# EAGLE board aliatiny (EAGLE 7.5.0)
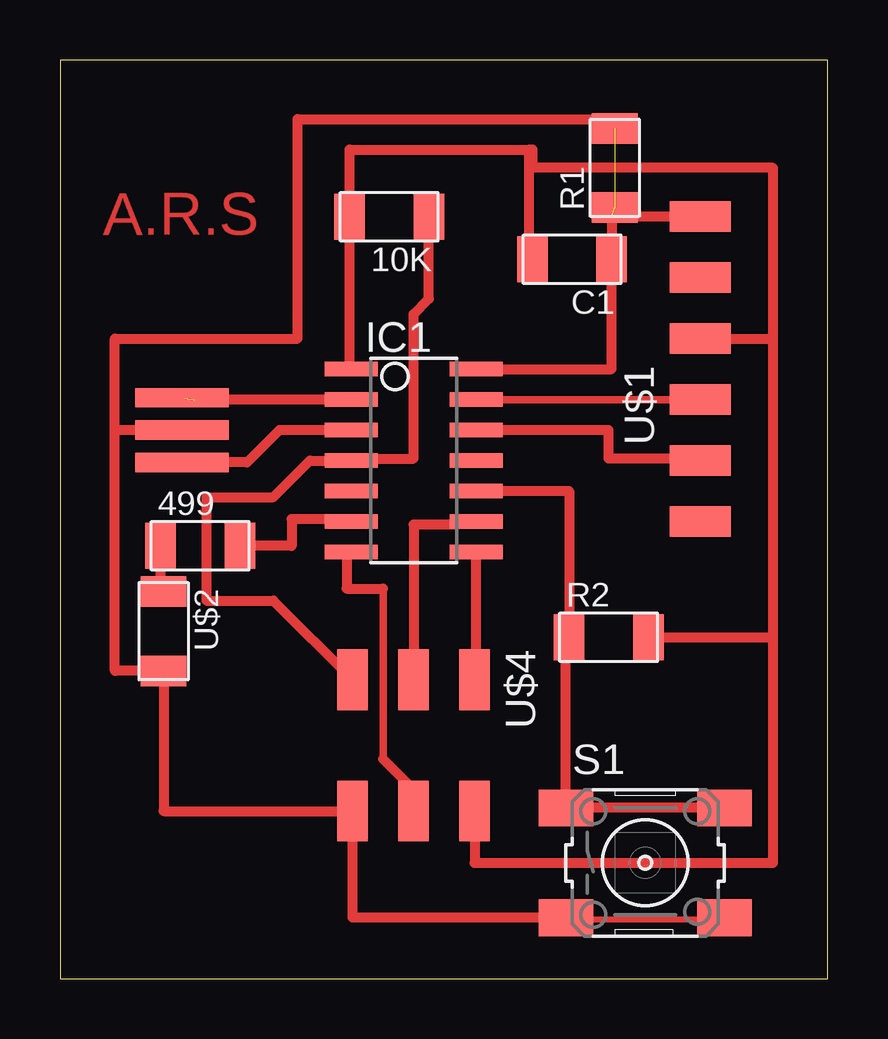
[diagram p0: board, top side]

Size 31.98 x 38.28 mm. Coordinates in mm from the lower left corner, seen from the top.
Outline: 0,0 31.98,0 31.98,38.28 0,38.28 0,0
Copper layers (1*16): Top 0.035mm / dielectric 1.5mm / Bottom 0.035mm
Design rules "default": minimum track width 10mil, minimum drill 24mil, track to track 8mil, track to pad 8mil, pad to pad 8mil, via to via 8mil, smd to smd 8mil, copper to edge 40mil, drill to drill 8mil, minimum pad ring 10mil, minimum via ring 8mil, stop-mask expansion 4mil, vias tented up to drill 0mil, thermal gap 10mil

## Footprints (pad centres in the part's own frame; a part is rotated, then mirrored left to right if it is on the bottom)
R1206FAB = smd 1.27 x 1.905: 1 -1.651,0; 2 1.651,0
C1206FAB = smd 1.27 x 1.905: 1 -1.651,0; 2 1.651,0
SOIC14 = smd 0.61 x 2.21: 1 -3.81,-2.603; 2 -2.54,-2.603; 3 -1.27,-2.603; 4 0,-2.603; 5 1.27,-2.603; 6 2.54,-2.603; 7 3.81,-2.603; 8 3.81,2.603; 9 2.54,2.603; 10 1.27,2.603; 11 0,2.603; 12 -1.27,2.603; 13 -2.54,2.603; 14 -3.81,2.603
6MM_SWITCH = smd 2.286 x 1.524: 1 -3.302,2.286; 2 3.302,2.286; 3 -3.302,-2.286; 4 3.302,-2.286
1X06SMD = smd 2.54 x 1.27: 1 0,6.35; 2 0,3.81; 3 0,1.27; 4 0,-1.27; 5 0,-3.81; 6 0,-6.35
LED1206FAB = smd 1.27 x 1.905: 1 -1.651,0; 2 1.651,0
EFOBM = smd 0.8 x 3.9: 1 -1.35,0; 2 0,0; 3 1.35,0
2X03SMD = smd 2.54 x 1.27: 1 -2.54,2.54; 2 2.92,2.54; 3 -2.54,0; 4 2.92,0; 5 -2.54,-2.54; 6 2.92,-2.54

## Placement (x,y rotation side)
10K  R  [R1206FAB]  13.72,31.75 180 top
499  [R1206FAB]  5.84,18.03 0 top
C1  [C1206FAB]  21.34,29.97 180 top
IC1  ATTINY44-SSU  [SOIC14]  14.73,21.59 270 top
R1  [R1206FAB]  23.11,33.78 90 top
R2  10k  [R1206FAB]  22.86,14.22 0 top
S1  [6MM_SWITCH]  24.38,4.83 0 top
U$1  FTDI-SMD-HEADER  [1X06SMD]  26.67,25.4 0 top
U$2  LEDFAB1206  [LED1206FAB]  4.32,14.48 270 top
U$3  RESONATOR  [EFOBM]  5.08,22.86 270 top
U$4  AVRISPSMD  [2X03SMD]  14.73,9.91 270 top

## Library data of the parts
10K 499 C1 IC1 R1 R2 S1 U$1-U$4 = fab

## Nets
BUTTON: IC1.10 R2.1 S1.1 S1.2
CTS: U$1.2
GND: C1.1 IC1.14 R1.1 R1.2 S1.3 S1.4 U$1.1 U$2.2 U$3.2 U$4.6
LED: 499.2 IC1.6
MISO: IC1.8 U$4.1
MOSI: IC1.7 U$4.4
N$4: IC1.2 U$3.1
N$5: IC1.3 U$3.3
N$6: 499.1 U$2.1
RST: 10K.1 IC1.4 U$4.5
RTS: U$1.6
RXD: IC1.12 U$1.5
SCK: IC1.9 U$4.3
TXD: IC1.13 U$1.4
VCC: 10K.2 C1.2 IC1.1 R2.2 U$1.3 U$4.2

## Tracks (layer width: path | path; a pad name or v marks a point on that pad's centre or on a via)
BUTTON
  Top 0.406: S1.2 S1.1 21.08,14.22 R2.1 21.21,20.32 IC1.10
GND  (2 unrouted)
  Top 0.254: S1.3 21.21,2.46 27.61,2.46 S1.4
  Top 0.406: S1.3 12.19,2.54 U$4.6 4.32,6.99 U$2.2 2.29,12.83 2.29,22.86 | IC1.14 22.99,25.4 C1.1 22.99,31.75 U$1.1 | U$3.2 2.29,22.86 | 2.29,22.86 2.29,26.67 9.91,26.67 9.91,35.81 22.86,35.81 22.86,35.43 R1.2
LED
  Top 0.254: 12.06,19.15 IC1.6
  Top 0.406: 12.06,19.15 9.65,19.15 9.65,18.03 499.2
MISO
  Top 0.254: IC1.8 | 17.32,12.52 U$4.1
  Top 0.406: 17.32,12.52 17.34,12.52 IC1.8
MOSI
  Top 0.305: 13.46,16.26 13.46,9.14
  Top 0.406: IC1.7 11.94,17.78 11.94,16.26 13.46,16.26 | U$4.4 14.73,7.87 13.46,9.14
N$4  (1 unrouted)
  Top 0.254: 12.06,24.18 IC1.2 | 5.21,24.18 U$3.1
  Top 0.406: 12.06,24.18 12.01,24.13 5.59,24.13
N$5
  Top 0.254: 12.06,22.81 IC1.3 | 5.21,21.67 U$3.3
  Top 0.406: 12.06,22.81 12.01,22.86 9.14,22.86 7.79,21.51 U$3.3
N$6
  Top 0.406: U$2.1 4.19,16.13 499.1
RST
  Top 0.254: 12.98,21.67 12.29,21.67 IC1.4 | 15.27,31.73 10K.1
  Top 0.406: U$4.5 8.89,15.75 6.1,15.75 6.1,20.07 8.89,20.07 10.41,21.59 IC1.4 | 12.98,21.67 14.73,21.67 14.73,27.69 15.37,28.32 10K.1
RXD
  Top 0.254: 17.55,22.81 IC1.12 | 26.47,21.67 U$1.5
  Top 0.406: 26.47,21.67 22.86,21.67 22.86,22.86 IC1.12
SCK
  Top 0.254: 16.41,18.92 17.32,18.92 IC1.9 | 14.81,12.52 U$4.3
  Top 0.406: 16.41,18.92 14.73,18.92 U$4.3
TXD
  Top 0.254: 17.55,24.18 IC1.13 | 26.47,24.18 U$1.4
  Top 0.305: 17.6,24.13 U$1.4
  Top 0.406: 17.55,24.18 17.6,24.13
VCC
  Top 0.254: 12.06,25.55 IC1.1
  Top 0.406: U$4.2 17.27,4.83 29.72,4.83 29.72,14.22 | 29.72,14.22 29.72,26.67 | R2.2 29.72,14.22 | U$1.3 29.72,26.67 | 29.72,26.67 29.72,33.78 19.69,33.78 19.69,34.54 19.56,34.54 | 19.56,34.54 12.06,34.54 10K.2 12.06,25.55 | C1.2 19.56,29.97 19.56,34.54

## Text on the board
Top: A.R.S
